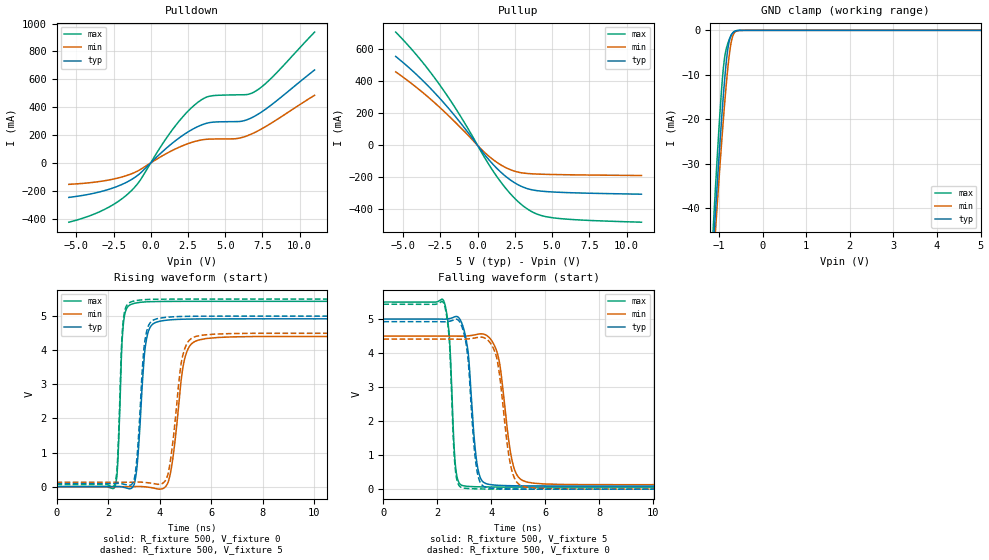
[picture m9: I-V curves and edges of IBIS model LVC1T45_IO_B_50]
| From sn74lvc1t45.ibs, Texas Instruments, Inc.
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[Model]   LVC1T45_IO_B_50
Model_type  I/O
Vinl=1.35
Vinh=3.85
Enable   Active-Low
Vref =   0
Rref =   2000
Cref =   15p
Vmeas =   2.5
| variable   typ   min   max
C_comp   6.40pF   5.43pF   7.92pF
| C_pullup   10.12pF   8.52pF   12.70pF
| C_pulldown   8.71pF   6.85pF   10.92pF
| C_tri-state   6.40pF   5.43pF   7.92pF
[Temperature Range]   40   100   -40
| Ambient temperature   25   85   -40
[Voltage range]   5   4.5   5.5
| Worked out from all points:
|   slope of the pulldown table from 0 to 0.75 V, typ, clamps not added: 9.75 ohm
|   slope of the pullup table from 0 to 0.75 V, typ, clamps not added: 8.46 ohm
|   GND clamp passes 1 mA (typ) near -0.71 V on its own axis
|   rising waveform, R_fixture 500, V_fixture 0: 20-80 % time 252ps typ, 390ps min, 153ps max; typ from 0 V to 4.92 V
|   falling waveform, R_fixture 500, V_fixture 5: 20-80 % time 277ps typ, 406ps min, 178ps max; typ from 5 V to 0.092 V
|   rising waveform, R_fixture 500, V_fixture 5: 20-80 % time 243ps typ, 377ps min, 152ps max; typ from 0.092 V to 5 V
|   falling waveform, R_fixture 500, V_fixture 0: 20-80 % time 275ps typ, 397ps min, 172ps max; typ from 4.92 V to 0 V
[GND Clamp]
| LVC1T45_IO_B_50
|   Voltage   I(typ)   I(min)   I(max)
-5.5V     -910.9mA   -836.3mA   -1.031A
-1.135V   -49.53mA   -53.14mA   -44.94mA
-1.12V    -47.12mA   -50.9mA    -42.25mA
-1.1V     -43.92mA   -47.92mA   -38.71mA
-1.07V    -39.19mA   -43.51mA   -33.49mA
-955mV    -22.02mA   -27.29mA   -15.21mA
-880mV    -12.18mA   -17.61mA   -6.789mA
-825mV    -6.376mA   -11.28mA   -3.86mA
-770mV    -2.643mA   -6.035mA   -2.191mA
-710mV    -920.7uA   -2.212mA   -923.3uA
-640mV    -245.9uA   -461.9uA   -195.8uA
5V        15.38pA    101.8nA    12.33pA
[Pulldown]
| LVC1T45_IO_B_50
|   Voltage   I(typ)   I(min)   I(max)
-5.5V     -247.8mA   -154.1mA   -425.7mA
-3.17V    -201.1mA   -129.5mA   -337.6mA
-1.43V    -128.1mA   -83.89mA   -213mA
-715mV    -75.2mA    -48.65mA   -125.8mA
1.54V     149mA      93.97mA    250mA
3.14V     259.4mA    158.6mA    432.6mA
3.99V     289.7mA    170.6mA    479.4mA
5.81V     296.3mA    175mA      488.4mA
6.515V    311.6mA    196.1mA    491.3mA
7.04V     338.7mA    221.1mA    514.8mA
8.205V    424.9mA    292.7mA    619.5mA
11V       666.8mA    485.2mA    938.6mA
[Pullup]
| LVC1T45_IO_B_50
|   Voltage   I(typ)   I(min)   I(max)
-5.5V     556.3mA    459.8mA    708.3mA
-3.9V     425mA      347.2mA    543mA
-2.385V   278.3mA    224.1mA    357.5mA
-1.08V    132.9mA    105.2mA    172.2mA
260mV     -32.41mA   -24.88mA   -42.78mA
945mV     -109.3mA   -81.77mA   -146.9mA
2.04V     -204.9mA   -145.3mA   -285mA
3.085V    -261.6mA   -172.9mA   -380mA
3.975V    -282.4mA   -178.8mA   -428.7mA
5.03V     -290.8mA   -181.7mA   -451.9mA
7.055V    -297.7mA   -184.5mA   -466.8mA
11V       -304.7mA   -188mA     -479.7mA
[Ramp]
| LVC1T45_IO_B_50
| variable   typ   min   max
dV/dt_r   2.99/2.63E-10   2.69/4.00E-10   3.30/1.61E-10
dV/dt_f   2.99/2.91E-10   2.66/4.21E-10   3.32/1.85E-10
R_load = 500
[Rising Waveform]
| LVC1T45_IO_B_50
R_fixture =   500
C_fixture =   0
L_fixture =   0
V_fixture =   0
V_fixture_min = 0
V_fixture_max = 0
|   Time   V(typ)   V(min)   V(max)
0s        225.7pV    389.5pV    145.6pV
2.27ns    2.056mV    38.72uV    -7.174mV
2.595ns   -17.16mV   -92.79uV   4.758V
2.98ns    12.87mV    1.984mV    5.366V
3.455ns   4.14V      -5.988mV   5.417V
3.915ns   4.832V     -67.18mV   5.428V
4.365ns   4.887V     203.4mV    5.431V
4.955ns   4.91V      3.679V     5.433V
5.52ns    4.917V     4.3V       5.433V
24.99ns   4.92V      4.406V     5.433V
[Falling Waveform]
| LVC1T45_IO_B_50
R_fixture =   500
C_fixture =   0
L_fixture =   0
V_fixture =   5
V_fixture_min = 4.5
V_fixture_max = 5.5
|   Time   V(typ)   V(min)   V(max)
0s        5V         4.5V       5.5V
2.24ns    4.996V     4.5V       5.527V
2.44ns    5.011V     4.5V       4.536V
2.67ns    5.073V     4.498V     691.1mV
2.94ns    4.805V     4.496V     105.1mV
3.475ns   720.4mV    4.55V      70.03mV
3.85ns    152.1mV    4.506V     64.85mV
4.815ns   99.98mV    691.1mV    61.17mV
5.315ns   95.69mV    208.9mV    60.67mV
24.99ns   91.93mV    128.8mV    60.15mV
[Rising Waveform]
| LVC1T45_IO_B_50
R_fixture =   500
C_fixture =   0
L_fixture =   0
V_fixture =   5
V_fixture_min = 4.5
V_fixture_max = 5.5
|   Time   V(typ)   V(min)   V(max)
0s        91.89mV    128.7mV    60.13mV
2.27ns    93.94mV    128.7mV    67.39mV
2.585ns   76.47mV    128.6mV    4.824V
2.955ns   101.7mV    130.4mV    5.432V
3.425ns   4.24V      124.6mV    5.483V
3.86ns    4.914V     77.89mV    5.494V
4.325ns   4.969V     351.4mV    5.498V
4.875ns   4.99V      3.756V     5.499V
5.435ns   4.997V     4.41V      5.5V
24.99ns   5V         4.5V       5.5V
[Falling Waveform]
| LVC1T45_IO_B_50
R_fixture =   500
C_fixture =   0
L_fixture =   0
V_fixture =   0
V_fixture_min = 0
V_fixture_max = 0
|   Time   V(typ)   V(min)   V(max)
0s        4.923V     4.41V      5.435V
2.24ns    4.919V     4.41V      5.459V
2.435ns   4.932V     4.41V      4.475V
2.66ns    4.991V     4.408V     624.1mV
2.91ns    4.776V     4.405V     44.55mV
3.45ns    629.5mV    4.453V     9.068mV
3.815ns   52.93mV    4.416V     4.396mV
4.755ns   6.967mV    563.1mV    994.9uV
5.23ns    3.351mV    67.88mV    527.3uV
24.99ns   36.9uV     71.58uV    18.7uV
